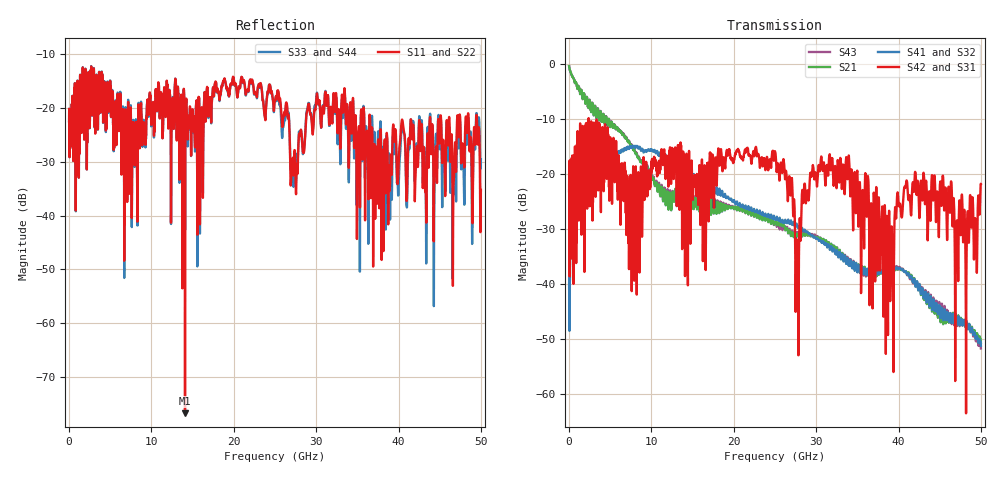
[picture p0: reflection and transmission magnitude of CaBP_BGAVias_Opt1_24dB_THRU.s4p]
!* Samtec Inc. NovaRay Examax Flyover System  *
!*  REV DATE  = 08/08/18  *
!*  TYPE  = TOUCHSTONE  *
!*  PORTS  = 4 port  *
!*  UNITS  = GHz  *
!*  DATA RANGE = DC  to 50 GHz; 10 MHz Step  *
!*  PARAMETER  = S  *
!*  FORMAT  = Real-Imaginary  *
!*  REFERENCE  = 50 ohms  *
!*  SOURCE  = HFSS  *
!*  VALIDATED  = No  *
!*  MANUFACTURER = SAMTEC  *
!*  INTERCONNECT = NVAx to EBCx to EBCx to NVAx  *
!*  [Full Channel NVAx to EBCx to EBCx to NVAx  with PCB Trace and BGA Via]  *
!*  BOUNDARY A  = Silicon BGA Ball Pad  *
!*  BOUNDARY B  = Silicon BGA Ball Pad  *
!*  NVAx (end a) ->>- (end b) NVAx  *
!*  Port 01 ->>- Port 02  *
!*  Port 03 ->>- Port 04  *
!***************************** CHANNEL MODEL ******************************************
# GHz S RI R 50
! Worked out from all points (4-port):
!   5000 points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, 10 MHz to 50 GHz, reference 50 ohm
!   strongest paths, dB at 10 MHz, 12.51 GHz, 25.01 GHz, 37.51 GHz, 50 GHz:
!     S42: -23.1, -15.2, -15.9, -27.7, -21.8
!     S31: -23.1, -15.2, -15.9, -27.7, -21.8
!     S41: -40.7, -18.2, -28.2, -37.9, -51.2
!     S32: -40.7, -18.2, -28.2, -37.9, -51.2
!     S21: -0.4, -24.1, -28.6, -38.2, -50.7
!     S43: -0.4, -24.0, -28.7, -37.9, -51.7
!   lowest |S11| = -76.8 dB at 14.08 GHz (marker M1), VSWR 1.00, Z = 50 - j0.00989 ohm
!   |S11| at or under -10 dB: start of sweep to end of sweep
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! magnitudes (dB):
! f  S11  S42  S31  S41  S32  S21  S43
! 10 MHz  -22.4  -23.1  -23.1  -40.7  -40.7  -0.4  -0.4
! 1.8 GHz  -17.1  -19.3  -19.3  -18.2  -18.2  -5.5  -5.5
! 14.08 GHz  -76.8  -38.5  -38.5  -18.7  -18.7  -26.0  -26.5
! 24.87 GHz  -20.5  -17.6  -17.6  -27.6  -27.6  -29.2  -29.2
! 27.69 GHz  -31.0  -32.7  -32.7  -29.4  -29.4  -31.0  -30.7
! 30.49 GHz  -20.3  -19.0  -19.0  -31.9  -31.9  -31.5  -31.5
! 50 GHz  -35.2  -21.8  -21.8  -51.2  -51.2  -50.7  -51.7
